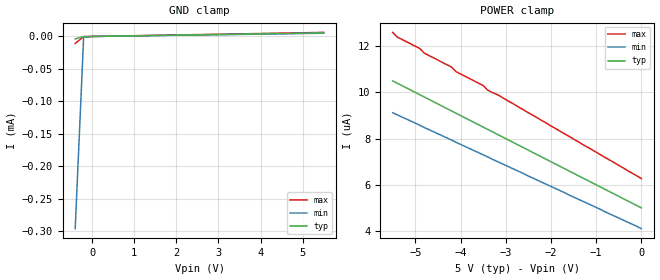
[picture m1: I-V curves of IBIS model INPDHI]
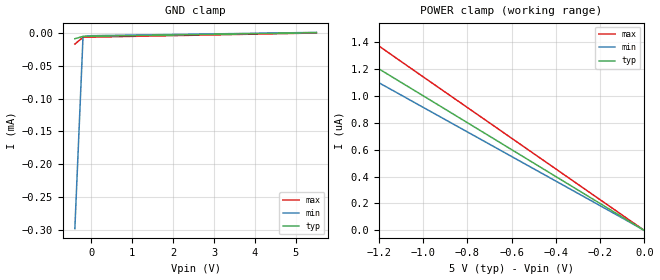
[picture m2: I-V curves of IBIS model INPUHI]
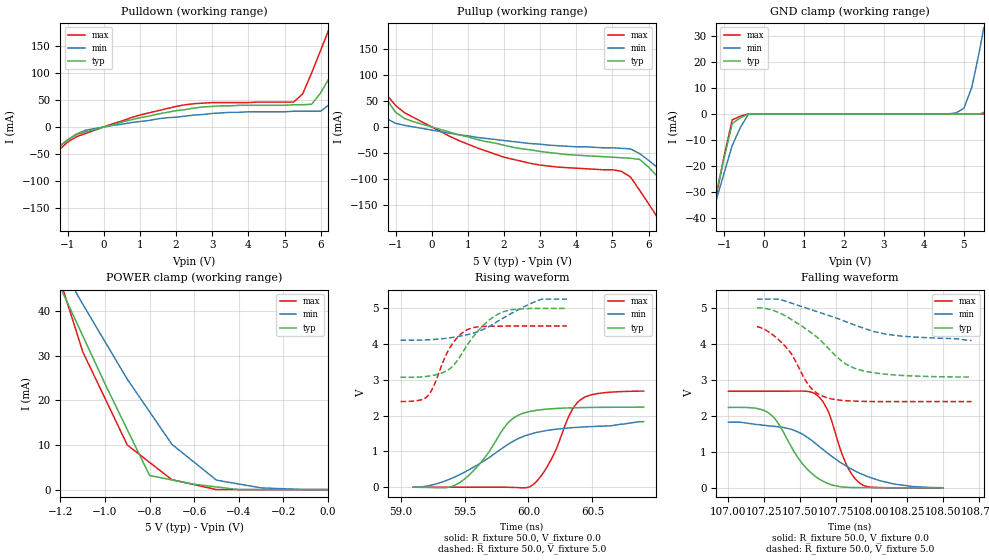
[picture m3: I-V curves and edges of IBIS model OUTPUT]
|   Texas Instruments Incorporated
|   Data Transmissions Products
|   IBIS Model for ISO723x4x
|   16DW SOIC Package
[IBIS Ver]   3.2
[Comment char]   |_char
[File name]   iso7240cf_5.ibs
[File Rev]   1.0
[Date]   10July08
[Source]   File originated at Texas Instruments Incorporated.
   Data Transmission Products Group.
[Notes]
[Disclaimer]
(C) Copyright Texas Instruments Incorporated 2002
   All rights reserved
  Texas Instruments Incorporated hereby grants the user of this IBIS
model a non-exclusive, nontransferable license to use this IBIS model
under the following terms.  Before using this IBIS model, the user
should read this license.  If the user does not accept these terms,
the IBIS model should be returned to Texas Instruments within 30 days.
  The user is granted this license only to use the IBIS model and
is not granted rights to sell, load, rent, lease or license the IBIS
model in whole or in part, or in modified form to anyone other than
user.  User may modify the IBIS model to suit its specific applications
but rights to derivative works and such modifications shall belong to
Texas Instruments.
  This IBIS model is provided on an "AS IS" basis and Texas Instruments
makes absolutely no warranty with respect to the information contained
herein.  TEXAS INSTRUMENTS DISCLAIMS AND CUSTOMER WAIVES ALL WARRANTIES,
EXPRESS OR IMPLIED, INCLUDING WARRANTIES OF MERCHANTABILITY OR FITNESS
FOR A PARTICULAR PURPOSE. The entire risk as to quality and performance
is with the Customer. ACCORDINGLY, IN NO EVENT SHALL THE COMPANY BE LIABLE
FOR ANY DAMAGES, WHETHER IN CONTRACT OR TORT,INCLUDING ANY LOST PROFITS
OR OTHER INCIDENTAL, CONSEQUENTIAL, EXEMPLARY, OR PUNITIVE DAMAGES ARISING
OUT OF THE USE OR APPLICATION OF THE IBIS model provided in this package.
Further, Texas Instruments reserves the right to discontinue or make changes
without notice to any product herein to improve reliability, function, or
design. Texas Instruments does not convey any license under patent rights
or any other intellectual property rights, including those of third parties.
Contact Texas Instruments at ATTN:DATA TRANSMISSIONS
[Copyright]   Copyright 2002, Texas Instruments, All Rights Reserved
[Component]   ISO7240DW
[Manufacturer]  Texas Instruments Incorporated
[Package]
|   typ   min   max
R_pkg   0.04817   0.03432   0.09530
L_pkg   2.4595nH   1.6904nH   4.7034nH
C_pkg   0.847pF   0.428pF   1.397pF
[Pin]   signal_name   model_name   R_pin   L_pin   C_pin
1   VCC1   POWER   0.03455  3.39778n  0.89677p
2   GND1   GND   0.03432  3.12613n  0.84706p
3   INA   INPUHI   0.04265  1.85523n  0.57831p
4   INB   INPUHI   0.03948  1.69049n  0.59300p
5   INC   INPUHI   0.03943  1.70546n  0.55709p
6   IND   INPUHI   0.04257  1.86953n  0.56379p
7   DISABLE   INPDHI   0.04783  1.99000n  0.60148p
8   GND1   GND   0.03740  4.70338n  1.39696p
9   GND2   GND   0.03763  4.61305n  1.39587p
10   CTRL   INPUHI   0.04703  2.01514n  0.58483p
11   OUTD   OUTPUT   0.07132  2.45946n  0.43321p
12   OUTC   OUTPUT   0.06147  2.13194n  0.42769p
13   OUTB   OUTPUT   0.07288  2.39260n  0.48001p
14   OUTA   OUTPUT   0.09530  3.03704n  0.47622p
15   GND2   GND   0.04817  4.23145n  0.93567p
16   VCC2   POWER   0.04790  4.51154n  0.99405p
| Models and submodels in the file (3): INPDHI (Input), INPUHI (Input), OUTPUT (3-state)
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|   Driver Enable
[Model]   INPDHI
Model_type   Input
|Signals   DISABLE
Vinh = 2.0
Vinl = 0.8
|   typ   min   max
C_comp   1.3pF   1.1pF   1.5pF
|   typ   min   max
[Temperature Range]   27   -40   85
[Voltage range]   5.0V   4.5V   5.5V
[GND_clamp]
|   Voltage   I(typ)   I(min)   I(max)
-400mV    -3.79uA    -296uA     -10.8uA
-200mV    -202nA     -1.2uA     -230nA
0V        0A         0A         0A
5.5V      5.5uA      5.02uA     6.27uA
[Power_clamp]
| Note that the[POWER_clamp]voltage table is referenced to Vcc
| and is calculated using Vtable=Vcc - Vmeasured.
|   Voltage   I(typ)   I(min)   I(max)
-5.5V     10.5uA     9.12uA     12.6uA
-5.4V     10.4uA     9.03uA     12.4uA
-4.9V     9.9uA      8.58uA     11.9uA
-4.8V     9.8uA      8.48uA     11.7uA
-4.2V     9.2uA      7.94uA     11.1uA
-4.1V     9.1uA      7.84uA     10.9uA
-3.5V     8.5uA      7.3uA      10.3uA
-3.4V     8.4uA      7.21uA     10.1uA
-3.1V     8.1uA      6.93uA     9.81uA
0V        5uA        4.1uA      6.27uA
|   Driver Input / Receiver Enable Model
[Model]   INPUHI
Model_type   Input
|Signals   INA,INB,INC,IND,EN
Vinh = 2.0
Vinl = 0.8
|   typ   min   max
C_comp   1.3pF   1.1pF   1.5pF
|   typ   min   max
[Temperature Range]   27   -40   125
[Voltage range]   5.0V   4.5V   5.5V
[GND_clamp]
|   Voltage   I(typ)   I(min)   I(max)
-400mV    -8.71uA    -298uA     -16.9uA
-200mV    -5.2uA     -5.27uA    -6.5uA
0V        -5uA       -4.1uA     -6.27uA
5.5V      500nA      913nA      27.5pA
[Power_clamp]
| Note that the[POWER_clamp]voltage table is referenced to Vcc
| and is calculated using Vtable=Vcc - Vmeasured.
|   Voltage   I(typ)   I(min)   I(max)
-5.5V     5.498uA    5.021uA    6.28uA
-1.7V     1.699uA    1.552uA    1.939uA
-1.6V     1.599uA    1.461uA    1.825uA
-1.5V     1.499uA    1.369uA    1.711uA
-1.4V     1.399uA    1.278uA    1.597uA
-1.3V     1.299uA    1.187uA    1.483uA
0V        0A         0A         0A
[Model]   OUTPUT
Model_type   3-state
| Signals   OUT
Vmeas = 2.2V   |Reference voltage for timing measurements
Cref = 15pF   |Timing specification test load capacitance value
Vref = 0   |Timing specification test load voltage; GND
| variable   typ   min   max
C_comp   2.1pF   1.7pF   2.5pF
|   typ   min   max
[Temperature Range]   25.0   -40   125
[Voltage range]   5.0V   5.5V   4.5V
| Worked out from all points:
|   slope of the pulldown table from 0 to 0.75 V, typ, clamps not added: 57.7 ohm
|   slope of the pullup table from 0 to 0.75 V, typ, clamps not added: 50 ohm
|   GND clamp passes 1 mA (typ) near -0.54 V on its own axis
|   POWER clamp passes 1 mA (typ) near -0.57 V on its own axis
|   rising waveform, R_fixture 50.0, V_fixture 0.0: 20-80 % time 272ps typ, 529ps min, 199ps max; typ from -0.001 V to 2.23 V
|   falling waveform, R_fixture 50.0, V_fixture 0.0: 20-80 % time 221ps typ, 412ps min, 143ps max; typ from 2.24 V to 0 V
|   rising waveform, R_fixture 50.0, V_fixture 5.0: 20-80 % time 247ps typ, 360ps min, 162ps max; typ from 3.07 V to 4.99 V
|   falling waveform, R_fixture 50.0, V_fixture 5.0: 20-80 % time 348ps typ, 508ps min, 205ps max; typ from 5.01 V to 3.08 V
[Pulldown]
|   Voltage   I(typ)  I(min)  I(max)
-5.5V     -360mA     -275mA     -490mA
-4V       -244mA     -190mA     -329mA
-2.75V    -148mA     -119mA     -195mA
-1.25V    -37mA      -37mA      -43mA
-500mV    -9mA       -6mA       -12mA
2.25V     32mA       20mA       41mA
5.25V     41mA       29mA       46mA
5.75V     42mA       29mA       100mA
6.25V     92mA       42mA       184mA
7V        185mA      107mA      314mA
8V        312mA      199mA      490mA
11V       716mA      492mA      1.045A
[Pullup]
|   Voltage   I(typ)  I(min)  I(max)
| Note that the[Pullup]voltage table is referenced to Vcc
| and is calculated using Vtable=Vcc - Vmeasured.
-5.5V     585mA      403mA      786mA
-3.25V    301mA      193mA      396mA
-2.25V    175mA      101mA      224mA
-2V       144mA      78mA       182mA
-1.25V    53mA       16mA       62mA
-750mV    16mA       3mA        27mA
2V        -35mA      -26mA      -58mA
5.25V     -59mA      -41mA      -85mA
6.5V      -114mA     -92mA      -201mA
7.5V      -192mA     -149mA     -309mA
8.25V     -251mA     -192mA     -391mA
10.5V     -429mA     -322mA     -637mA
[GND_clamp]
|   Voltage   I(typ)   I(min)   I(max)
| Outputs in High Impedance (off)
-5.5V     -359.9mA   -275.1mA   -489.5mA
-1.4V     -44.92mA   -43.82mA   -51.83mA
-1.3V     -37.54mA   -38.38mA   -41.63mA
-1.2V     -30.16mA   -32.94mA   -31.43mA
-1V       -16.66mA   -22.42mA   -15.87mA
-800mV    -3.66mA    -12.05mA   -2.249mA
-600mV    -1.479mA   -5.279mA   -861.1uA
-400mV    -1.657uA   -187.7uA   -4.797uA
4.8V      37.53pA    388.9uA    31.79pA
5V        41.24pA    2.119mA    35.42pA
5.2V      2.711nA    10.13mA    39.28pA
5.5V      594.7uA    33.09mA    45.67pA
[POWER_clamp]
|   Voltage  I(typ)   I(min)   I(max)
| Note that the [POWER_clamp] voltage table is referenced to Vcc
| and is calculated using Vtable = Vcc - Vmeasured.
| Outputs in Tri-state.
-5.5V     585.2mA    450.6mA    785.6mA
-1.2V     45.19mA    50.27mA    46.63mA
-1.1V     34.43mA    41.5mA     30.85mA
-1V       23.66mA    33.09mA    20.41mA
-900mV    13.4mA     24.69mA    9.969mA
-800mV    3.151mA    17.41mA    6.092mA
-700mV    2.17mA     10.13mA    2.215mA
-600mV    1.189mA    6.126mA    1.108mA
-500mV    594.7uA    2.119mA    44.53nA
-400mV    8.158nA    1.254mA    22.74nA
-300mV    5.434nA    388.9uA    942.3pA
0V        41.24pA    132.3nA    45.67pA
[Ramp]
|   typ   min   max
dV/dt_r   1.341V/0.27ns   1.043V/0.48ns   1.610V/0.20ns
dV/dt_f   1.342V/0.22ns   1.044V/0.40ns   1.613V/0.14ns
R_load = 50
[Rising Waveform]
R_fixture = 50.0
V_fixture = 0.0
C_fixture = 0p
L_fixture = 0n
|   V(typ)   V(min)   V(max)
59.1ns    -971.8uV   -826.8uV   -150.2nV
59.46ns   123.7mV    348.7mV    -5.006uV
59.64ns   742.1mV    706.8mV    166.3uV
59.84ns   1.794V     1.197V     -2.714mV
60ns      2.104V     1.465V     -1.679mV
60.14ns   2.178V     1.582V     537.6mV
60.32ns   2.214V     1.656V     2.018V
60.4ns    2.221V     1.675V     2.421V
60.56ns   2.229V     1.703V     2.624V
60.9ns    2.234V     1.83V      2.683V
[Falling Waveform]
R_fixture = 50.0
V_fixture = 0.0
C_fixture = 0p
L_fixture = 0n
|   V(typ)   V(min)   V(max)
107ns     2.237V     1.827V     2.687V
107.3ns   2.088V     1.723V     2.688V
107.4ns   1.14V      1.628V     2.691V
107.6ns   345mV      1.263V     2.631V
107.7ns   187.2mV    1.07V      2.403V
107.7ns   85.02mV    884.2mV    1.888V
107.8ns   13.06mV    566.3mV    521.5mV
107.9ns   6.705mV    369.2mV    74.72mV
108.2ns   1.957mV    106.2mV    2.74mV
108.5ns   260.9uV    688.9uV    8.263uV
[Rising Waveform]
R_fixture = 50.0
V_fixture = 5.0
V_fixture_min = 5.5
V_fixture_max = 4.5
C_fixture = 0p
L_fixture = 0n
|   V(typ)   V(min)  V(max)
59ns      3.071V     4.103V     2.393V
59.16ns   3.077V     4.107V     2.438V
59.22ns   3.1V       4.116V     2.578V
59.38ns   3.293V     4.167V     3.86V
59.44ns   3.518V     4.199V     4.163V
59.52ns   3.964V     4.257V     4.394V
59.64ns   4.498V     4.395V     4.486V
59.8ns    4.892V     4.717V     4.496V
60.1ns    4.99V      5.245V     4.5V
60.3ns    4.99V      5.25V      4.5V
[Falling Waveform]
R_fixture = 50.0
V_fixture = 5.0
V_fixture_min = 5.5
V_fixture_max = 4.5
C_fixture = 0p
L_fixture = 0n
|   V(typ)   V(min)  V(max)
107.2ns   5.011V     5.25V      4.487V
107.3ns   4.956V     5.25V      4.288V
107.4ns   4.778V     5.191V     3.926V
107.4ns   4.684V     5.139V     3.731V
107.6ns   4.368V     4.98V      2.859V
107.7ns   3.961V     4.822V     2.518V
107.8ns   3.5V       4.654V     2.431V
107.9ns   3.258V     4.451V     2.406V
108.2ns   3.13V      4.225V     2.4V
108.7ns   3.081V     4.1V       2.4V
